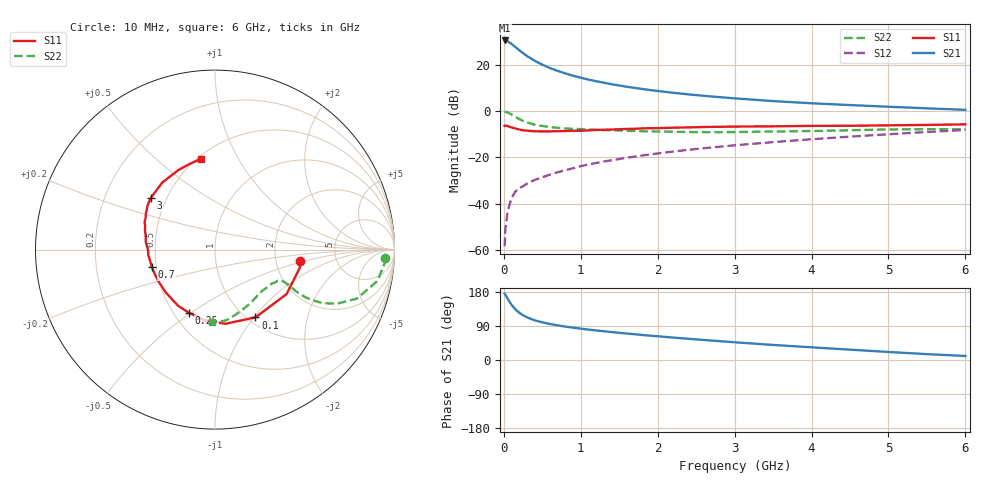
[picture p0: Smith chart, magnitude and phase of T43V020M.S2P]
! Infineon Technologies  Discrete & RF Semiconductors
! BFR182T
! Si NPN RF Bipolar Junction Transistor in SC75
! VCE = 3 V  IC = 20 mA
! Common Emitter S-Parameters:  October  1999
# GHz  S  MA  R  50
!  f  S11  S21  S12  S22
! GHz  MAG  ANG  MAG  ANG  MAG  ANG  MAG  ANG
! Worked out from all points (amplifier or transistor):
!   36 points, 10 MHz to 6 GHz, reference 50 ohm
!   highest |S21| = 30.4 dB at 10 MHz (marker M1)
!   |S21| within 3 dB of that: start of sweep to 156.2 MHz
!   unconditionally stable (mu >= 1): start of sweep to 10.27 MHz; 607.2 MHz to 3.665 GHz
!   at 250 MHz: K = 0.68, MSG = 28.7 dB, |S12| = -32.5 dB
!   at 1.4 GHz: K = 1.12, MAG = 14.3 dB, |S12| = -21.3 dB
!   at 6 GHz: K = 0.84, MSG = 4.3 dB, |S12| = -8.2 dB
!   S11 on the Smith chart (normalised r, x): 10 MHz: 2.73, -0.44; 100 MHz: 1.09, -1.02; 250 MHz: 0.60, -0.49; 700 MHz: 0.47, -0.10; 3 GHz: 0.41, +0.30; 6 GHz: 0.52, +0.72
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0.01  0.4757 -7.5  33.22 175.1  0.0012 76.0  0.9496 -2.8
0.02  0.4838 -11.8  33.2 172.4  0.0028 97.8  0.9495 -4.3
0.05  0.4697 -31.8  31.81 161.3  0.0069 83.0  0.9221 -10.9
0.1  0.4399 -59.2  27.99 145.8  0.0131 71.5  0.8355 -19.1
0.15  0.4173 -82.1  23.98 133.6  0.0182 65.1  0.7422 -24.0
0.2  0.3981 -98.7  20.49 124.7  0.0215 64.4  0.6674 -26.5
0.25  0.3812 -112.1  17.62 118.0  0.0237 63.3  0.6073 -27.5
0.3  0.3746 -123.3  15.37 112.7  0.0268 64.0  0.565 -27.8
0.4  0.3634 -139.3  12.14 104.8  0.0323 63.9  0.5048 -27.2
0.5  0.3616 -150.0  9.969 99.4  0.037 65.5  0.4721 -26.1
0.6  0.3622 -158.4  8.414 95.0  0.0422 66.8  0.4487 -25.5
0.7  0.3654 -164.8  7.308 91.4  0.0474 68.1  0.4315 -25.1
0.9  0.3731 -175.5  5.749 85.4  0.0578 70.3  0.409 -25.1
1.1  0.3806 176.6  4.755 80.2  0.0698 71.1  0.3968 -26.0
1.3  0.3916 170.3  4.059 75.8  0.0808 71.4  0.3855 -27.5
1.6  0.4081 162.9  3.322 69.8  0.0975 71.4  0.3724 -30.1
2.2  0.4339 152.6  2.464 59.2  0.1326 70.7  0.3556 -37.7
3  0.4587 141.1  1.867 46.8  0.181 68.1  0.3499 -49.0
3.5  0.4649 134.3  1.63 39.7  0.2118 66.0  0.3586 -57.0
4.5  0.4778 121.9  1.337 27.3  0.2785 60.7  0.3819 -73.1
5.5  0.4983 106.2  1.136 15.5  0.3503 54.4  0.4031 -86.7
6  0.5121 98.6  1.055 10.6  0.3879 50.4  0.4014 -92.4
